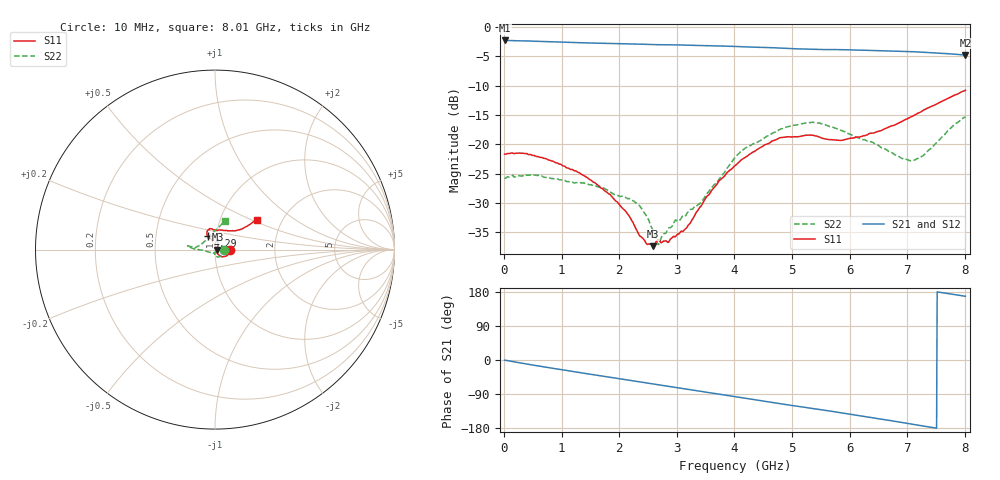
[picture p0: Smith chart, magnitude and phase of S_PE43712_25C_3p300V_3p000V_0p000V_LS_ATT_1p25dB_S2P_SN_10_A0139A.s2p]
! DEVICE ID: PE43712
! File Path: z:\PE43713\PE43713_CHAR_NOM_04292014\AMB\3p300\LS_ATT_1p25dB\PE43713_AMB_3p300V_3p000V_0p000V_LS_ATT_1p25dB_S2P_SN_10_A0139A.s2p
! Serial: 10
! Lot: A0139A
! Temp: 25C
! VDD: 3.300
! VSS: 0.000
! Control_Hi: 3.000
! Control_Lo: 0.000
! Attenuation Step: 1.25dB
! Port 1: RF1
! Port 2: RF2
! ThroughPath:1-2
! IDD: 0.0001469176
! ISS: -5.73e-008
#  Hz  S  RI  R  50
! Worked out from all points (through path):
!   801 points, 10 MHz to 8.01 GHz, reference 50 ohm
!   highest |S21| = -2.27 dB at 10 MHz (marker M1); lowest = -4.8 dB at 8.01 GHz (marker M2)
!   group delay of S21, straight-line fit = 65.7 ps
!   lowest |S11| = -37.4 dB at 2.59 GHz (marker M3), VSWR 1.03, Z = 51.4 + j0.0396 ohm
!   |S11| at or under -10 dB: start of sweep to end of sweep
!   |S22| runs from -37.1 to -15.3 dB; largest |S21 - S12| = 0.0023
!   S11 on the Smith chart (normalised r, x): 10 MHz: 1.18, -0.00; 4.29 GHz: 0.91, +0.14; 8.01 GHz: 1.50, +0.55
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1e7  0.0827 -0.000471  0.77 -0.00416  0.7699 -0.00405  0.0515 -0.000592
6.8e8  0.0696 -0.0315  0.7182 -0.2307  0.7178 -0.2306  0.0451 -0.0275
1.35e9  0.0386 -0.0395  0.6099 -0.4117  0.6095 -0.4115  0.0227 -0.041
1.86e9  0.0218 -0.0293  0.5038 -0.5217  0.5036 -0.5214  0.00867 -0.0379
2.14e9  0.0138 -0.0216  0.4373 -0.5723  0.4372 -0.572  -0.000301 -0.0346
2.28e9  0.0129 -0.0146  0.402 -0.5946  0.4021 -0.5942  -0.00035 -0.0319
2.47e9  0.0127 -0.00647  0.3523 -0.6205  0.3525 -0.6205  -0.00217 -0.0245
2.59e9  0.0135 0.000385  0.3206 -0.6339  0.3206 -0.634  -0.0024 -0.0183
2.68e9  0.0145 0.00516  0.2976 -0.6438  0.2978 -0.6436  0.000447 -0.014
2.86e9  0.0107 0.0102  0.2482 -0.6628  0.2482 -0.663  -0.00549 -0.0186
3.14e9  0.00282 0.0187  0.168 -0.6829  0.1681 -0.6827  -0.0174 -0.017
3.43e9  -0.00284 0.0301  0.084 -0.6912  0.0843 -0.6915  -0.0291 -0.0145
3.74e9  -0.0122 0.0478  -0.00428 -0.6915  -0.00359 -0.6914  -0.05 -0.00932
4.01e9  -0.0252 0.0608  -0.0818 -0.6801  -0.0813 -0.6799  -0.0772 -0.00243
4.29e9  -0.0392 0.0742  -0.1574 -0.6576  -0.1568 -0.6579  -0.0985 0.00291
4.79e9  -0.0427 0.1056  -0.2821 -0.6  -0.2817 -0.6002  -0.1338 0.0106
5.35e9  -0.0257 0.1168  -0.3974 -0.5113  -0.3972 -0.5107  -0.1529 0.0215
5.86e9  0.0115 0.1076  -0.489 -0.417  -0.4878 -0.417  -0.1302 0.0161
6.68e9  0.0938 0.1045  -0.5853 -0.2221  -0.5852 -0.2218  -0.0838 0.0238
7.02e9  0.1271 0.1083  -0.6048 -0.132  -0.6043 -0.1323  -0.0561 0.0474
7.16e9  0.1422 0.1129  -0.6082 -0.0943  -0.6073 -0.0942  -0.0413 0.0627
8.01e9  0.2361 0.1674  -0.566 0.1189  -0.5643 0.1179  0.0573 0.1621
